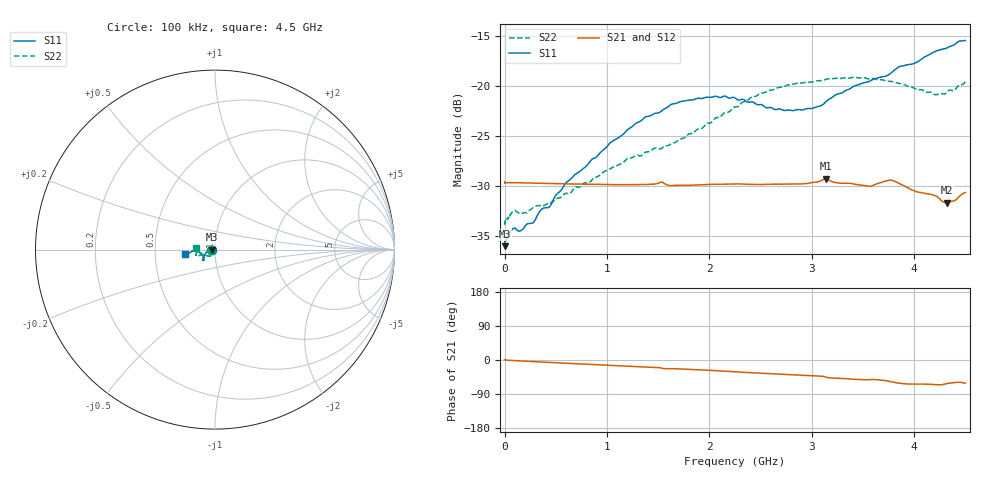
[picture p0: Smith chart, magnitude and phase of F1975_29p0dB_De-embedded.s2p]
! Integrated Device Technology
! Corporate Headquarters
! 6024 Silver Creek Valley Road
! San Jose, CA 95138  USA
! Phone:  1-408-284-8200
! Toll Free:  1-800-223-1366
! Webpage:  http://www.idt.com/
! Timing and RF Division
! 515 Groton Road, Suite 102
! Westford, MA 01886-6024
! Device:  F1975
! Description: 6-bit, 75 ohm, 0.5 dB Digital Step Attenuator
! Frequency:  5.0 MHz -  3.00 GHz
! Package:  4x4 mm QFN Plastic Package: 20 pin
! Ports:  2 RF, 11 DC
!  Pin  1  = D5 (16 dB)
!  Pin  2  = RF1  =  Port 1
!  Pin  3  = Serial Data In (DATA)
!  Pin  4  = Serial Clock (CLK)
!  Pin  5  = Serial Latch Enable (LE)
!  Pin  6  = VDD
!  Pin  7  = NC
!  Pin  8  = NC
!  Pin  9  = NC
!  Pin 10  = GND
!  Pin 11  = GND
!  Pin 12  = NC
!  Pin 13  = VMODE
!  Pin 14  = RF2  =  Port 2
!  Pin 15  = D4 (8 dB)
!  Pin 16  = D3 (4 dB)
!  Pin 17  = D2 (2 dB)
!  Pin 18  = NC
!  Pin 19  = D1 (1 dB)
!  Pin 20  = D0 (0.5 dB)
! State:  58
! Atten State:  29.0 dB
! Voltage:  +3.30 Volts
! Current:  0.592 mA
! Data:  The device was measured on a F1975 evaluation board which has
!  individual transmission lines to the RF pins.  Data was collected
!  using a calibrated network analyzer.  The evaluation board was
!  de-embedded using Automatic Fixture Removal (AFR).
!  The reference plane is the edge of the package pin.
! Misc:
!  Action Tracker AT0415
! Date Measured:  2018-02-08
! Date:  2018-03-26  MJV
! Note:
!  Integrated Device Technology supplies this data as a sample of measured
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# GHz S dB R 75
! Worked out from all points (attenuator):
!   291 points, 100 kHz to 4.5 GHz, reference 75 ohm
!   highest |S21| = -29.24 dB at 3.14 GHz (marker M1); lowest = -31.7 dB at 4.32 GHz (marker M2)
!   lowest |S11| = -36.0 dB at 100 kHz (marker M3), VSWR 1.03, Z = 72.7 - j0.00454 ohm
!   |S11| at or under -10 dB: start of sweep to end of sweep
!   |S22| runs from -33.9 to -19.1 dB; largest |S21 - S12| = 0.00013
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0.0001  -35.99 -179.9  -29.62 1.2  -29.60 1.2  -33.85 -179.0
0.005  -35.49 -178.0  -29.63 0.5  -29.63 0.5  -33.49 -177.6
0.08  -34.25 -176.5  -29.65 -1.2  -29.64 -1.2  -32.49 -169.5
0.16  -34.43 -177.9  -29.66 -2.5  -29.66 -2.5  -32.77 -160.0
0.28  -33.67 179.2  -29.69 -4.2  -29.69 -4.2  -32.12 -151.9
0.36  -32.32 179.2  -29.71 -5.4  -29.71 -5.4  -31.90 -144.4
0.44  -32.06 179.8  -29.73 -6.4  -29.72 -6.5  -31.81 -138.9
0.6  -29.65 -176.7  -29.77 -8.7  -29.77 -8.7  -30.70 -132.8
0.76  -28.31 -170.0  -29.79 -10.8  -29.80 -10.8  -29.81 -128.9
1.28  -23.73 -153.3  -29.85 -17.4  -29.84 -17.4  -26.92 -124.7
1.52  -22.59 -145.9  -29.63 -20.6  -29.63 -20.6  -26.28 -131.1
1.64  -21.78 -143.0  -29.94 -22.8  -29.93 -22.9  -25.69 -135.1
1.88  -21.23 -139.0  -29.88 -25.5  -29.87 -25.5  -24.33 -147.2
2.26  -21.25 -137.2  -29.78 -31.2  -29.78 -31.2  -22.07 -158.0
2.64  -22.35 -147.5  -29.80 -36.6  -29.80 -36.6  -20.32 -159.4
3.02  -22.17 -164.3  -29.62 -41.7  -29.61 -41.7  -19.54 -160.0
3.14  -21.53 -167.0  -29.24 -45.4  -29.24 -45.5  -19.31 -160.4
3.56  -19.53 -177.4  -30.01 -52.0  -30.01 -52.0  -19.29 -165.9
3.76  -18.80 -175.8  -29.39 -56.5  -29.39 -56.5  -19.53 -169.5
4.2  -16.56 -172.5  -30.93 -64.9  -30.93 -65.0  -20.85 179.0
4.32  -16.18 -172.0  -31.66 -62.3  -31.65 -62.3  -20.63 176.6
4.5  -15.44 -171.6  -30.64 -61.3  -30.63 -61.3  -19.57 173.9
